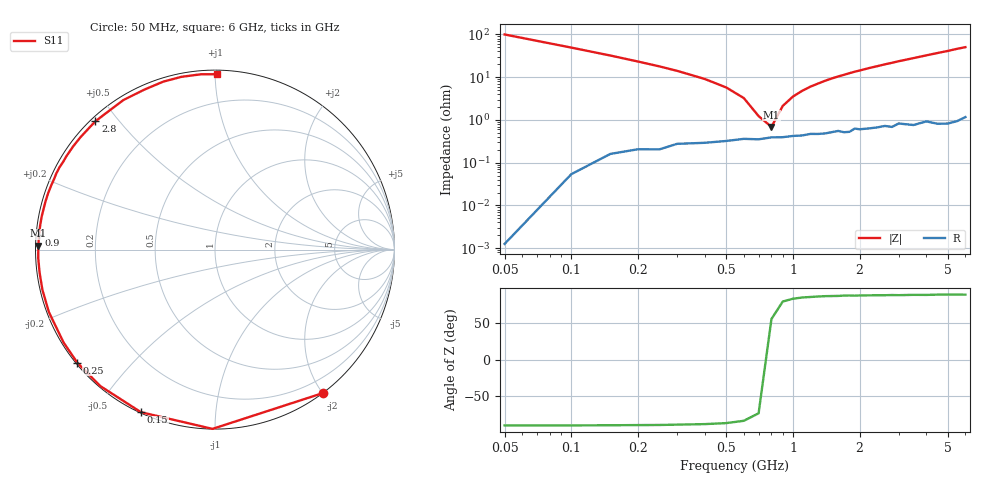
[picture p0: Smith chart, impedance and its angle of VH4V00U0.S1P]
! Infineon Technologies  Discrete & RF Semiconductors
! BB 814
! Si Tuning Diode in SOT23
! VR = 4 V
! S-Parameters:  July  1999
# GHz  S  MA  R  50
!  f  S11
! GHz  MAG  ANG
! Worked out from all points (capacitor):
!   34 points, 50 MHz to 6 GHz, reference 50 ohm
!   read as one part to ground: C = 31.7 pF near 50 MHz
!   lowest |Z| = 689 mohm at 800 MHz (marker M1)
!   series resonance near 767.5 MHz, so ESL is about 1.4 nH
!   S11 on the Smith chart (normalised r, x): 50 MHz: 0.00, -2.00; 150 MHz: 0.00, -0.64; 250 MHz: 0.00, -0.36; 900 MHz: 0.01, +0.04; 2.8 GHz: 0.01, +0.43; 6 GHz: 0.02, +1.01
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0.05  1 -53.1
0.1  0.9989 -90.8
0.15  0.9955 -114.5
0.2  0.9932 -130.1
0.25  0.9928 -140.6
0.3  0.9898 -148.5
0.4  0.9888 -159.4
0.5  0.9874 -166.9
0.6  0.9857 -172.6
0.7  0.986 -177.3
0.8  0.9845 178.7
0.9  0.9844 175.2
1  0.9834 172.0
1.2  0.9816 166.3
1.4  0.9813 161.2
1.6  0.979 156.5
1.7  0.9806 154.4
1.9  0.9769 149.9
2.2  0.9774 143.9
2.4  0.9766 140.2
2.8  0.9772 133.0
3  0.9734 129.4
3.5  0.9771 121.5
4  0.9744 114.0
4.5  0.9792 107.1
5  0.9806 101.0
5.5  0.98 94.6
6  0.9772 89.4
